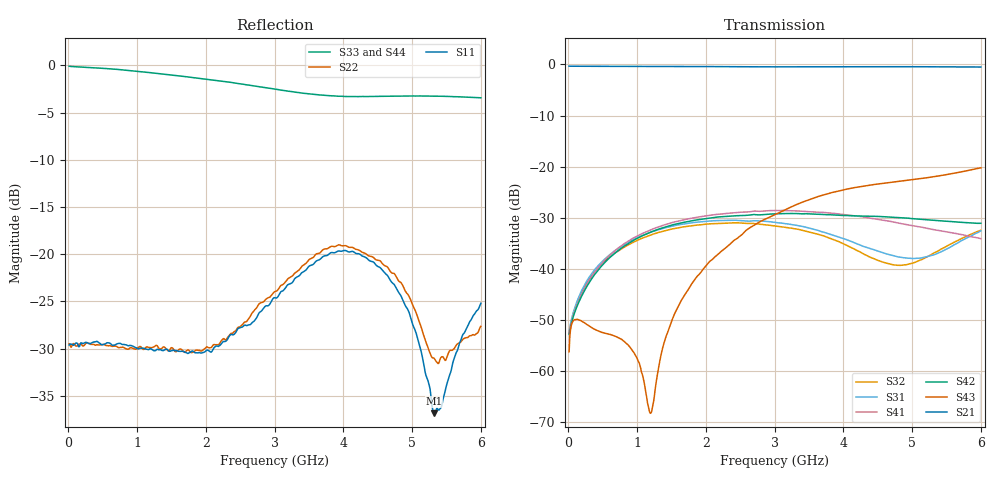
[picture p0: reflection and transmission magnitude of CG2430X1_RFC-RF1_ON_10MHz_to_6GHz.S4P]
!CEL
!CG2430X1
!Port1: RFC Port2: RF1  Port3: RF2 Port4: RF3
!Data & Calibration Information:
!Freq	S11:SOLT4(ON)	S12:SOLT4(ON)	S13:SOLT4(ON)	S14:SOLT4(ON)
!	S21:SOLT4(ON)	S22:SOLT4(ON)	S23:SOLT4(ON)	S24:SOLT4(ON)
!	S31:SOLT4(ON)	S32:SOLT4(ON)	S33:SOLT4(ON)	S34:SOLT4(ON)
!	S41:SOLT4(ON)	S42:SOLT4(ON)	S43:SOLT4(ON)	S44:SOLT4(ON)
# Hz S dB R 50
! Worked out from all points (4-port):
!   600 points, 10 MHz to 6 GHz, reference 50 ohm
!   strongest paths, dB at 10 MHz, 1.51 GHz, 3.01 GHz, 4.51 GHz, 6 GHz:
!     S21: -0.3, -0.4, -0.5, -0.4, -0.5
!     S43: -56.3, -50.0, -29.4, -23.4, -20.2
!     S42: -52.9, -31.4, -29.2, -29.8, -31.1
!     S41: -52.5, -31.0, -28.6, -30.4, -34.1
!     S31: -52.3, -31.7, -30.9, -36.6, -32.6
!     S32: -52.7, -32.2, -31.6, -38.4, -32.4
!   lowest |S11| = -36.8 dB at 5.32 GHz (marker M1), VSWR 1.03, Z = 51.3 - j0.586 ohm
!   |S11| at or under -10 dB: start of sweep to end of sweep
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1e7  -29.61 0.2  -0.34 -0.1  -52.36 13.2  -52.65 11.5
     -0.33 -0.2  -29.49 -1.6  -52.77 13.7  -52.98 11.6
     -52.33 14.4  -52.67 14.8  -0.07 -0.6  -56.34 53.2
     -52.49 12.1  -52.88 12.3  -56.26 52.2  -0.12 -0.4
1.2e9  -30.02 -5.9  -0.38 -9.5  -32.86 45.9  -32.35 54.2
       -0.39 -9.5  -29.89 -1.3  -33.38 51.2  -32.85 49.7
       -32.85 45.9  -33.38 51.0  -0.77 -50.5  -68.32 -77.5
       -32.36 53.9  -32.82 49.8  -68.26 -76.5  -0.68 -50.4
1.62e9  -30.29 -9.2  -0.39 -12.6  -31.37 38.4  -30.63 47.0
        -0.40 -12.6  -30.04 -6.2  -31.92 45.6  -31.07 41.3
        -31.36 38.3  -31.92 45.4  -1.11 -67.0  -46.76 -173.0
        -30.58 46.5  -31.07 41.4  -46.78 -173.2  -1.03 -67.0
2.59e9  -27.56 32.2  -0.44 -19.9  -30.68 23.1  -28.94 32.3
        -0.44 -19.9  -27.13 34.8  -31.18 33.9  -29.53 25.3
        -30.67 23.2  -31.13 34.1  -2.05 -100.5  -32.44 156.4
        -28.90 32.8  -29.55 25.4  -32.42 156.4  -1.92 -100.6
4.23e9  -19.96 47.0  -0.45 -32.1  -35.39 16.1  -29.77 8.6
        -0.46 -32.1  -19.58 44.2  -36.70 32.3  -29.71 7.2
        -35.28 15.6  -36.62 31.4  -3.30 -167.3  -23.95 100.9
        -29.74 8.5  -29.68 7.1  -23.95 100.7  -3.13 -164.2
5.32e9  -36.85 -23.4  -0.45 -41.5  -37.20 70.7  -32.43 -1.2
        -0.46 -41.5  -31.02 -28.3  -36.75 99.8  -30.49 2.8
        -37.26 69.8  -36.90 98.7  -3.25 164.3  -21.98 76.7
        -32.36 -0.6  -30.51 3.1  -21.97 76.5  -3.13 168.8
6e9  -25.19 -133.8  -0.49 -47.6  -32.42 92.7  -33.86 -6.5
     -0.50 -47.6  -27.63 -130.6  -32.38 112.1  -31.07 6.1
     -32.56 92.7  -32.44 112.7  -3.42 150.9  -20.22 63.3
     -34.13 -5.7  -31.10 6.2  -20.23 63.5  -3.34 155.9
